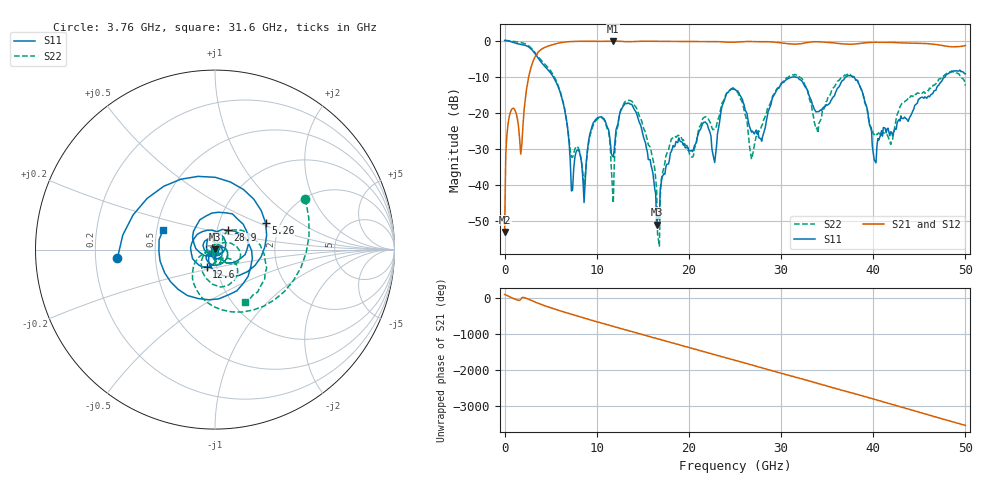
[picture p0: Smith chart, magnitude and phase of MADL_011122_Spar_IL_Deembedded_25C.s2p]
#	HZ	S	DB	R	50
!Frequency	S11 (dB)	S11-Ang	S21 Deemb (dB)	S21-Ang	S12 Deemb (dB)	S12-Ang	S22 (dB)	S22-Ang
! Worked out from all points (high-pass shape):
!   401 points, 10 MHz to 50 GHz, reference 50 ohm
!   highest |S21| = -0.15 dB at 11.8 GHz (marker M1); lowest = -53.1 dB at 10 MHz (marker M2)
!   |S21| within 3 dB of the highest: 3.681 GHz to end of sweep
!   lowest |S11| = -51.0 dB at 16.5 GHz (marker M3), VSWR 1.01, Z = 49.8 + j0.209 ohm
!   |S11| at or under -10 dB: 5.275 GHz to 37.1 GHz (31.83 GHz wide, 150 % of centre); 37.71 GHz to 47.82 GHz (10.1 GHz wide, 23.6 % of centre)
!   |S22| runs from -57.0 to 0.0 dB; largest |S21 - S12| = 0.017
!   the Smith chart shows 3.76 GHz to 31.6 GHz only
!   S11 on the Smith chart (normalised r, x): 3.76 GHz: 0.29, -0.04; 5.26 GHz: 1.67, +0.55; 12.6 GHz: 0.90, -0.17; 28.9 GHz: 1.12, +0.25; 31.6 GHz: 0.54, +0.13
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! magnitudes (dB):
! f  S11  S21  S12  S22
! 10 MHz  0.0  -53.1  -53.8  0.0
! 635 MHz  -0.3  -19.9  -19.9  -0.1
! 1.76 GHz  -1.1  -31.5  -31.5  -0.5
! 3.76 GHz  -5.3  -2.9  -2.9  -4.8
! 5.26 GHz  -9.9  -1.1  -1.1  -9.4
! 8.38 GHz  -34.2  -0.2  -0.2  -34.3
! 10.4 GHz  -21.2  -0.2  -0.2  -21.4
! 11.8 GHz  -32.3  -0.2  -0.1  -45.1
! 12.6 GHz  -19.5  -0.2  -0.2  -19.3
! 14.8 GHz  -23.7  -0.2  -0.2  -21.7
! 16.5 GHz  -51.0  -0.2  -0.2  -41.2
! 16.8 GHz  -49.7  -0.2  -0.2  -57.0
! 18.1 GHz  -30.8  -0.2  -0.2  -27.3
! 25.1 GHz  -13.8  -0.4  -0.4  -14.1
! 26.9 GHz  -25.1  -0.3  -0.3  -31.8
! 28.9 GHz  -17.8  -0.4  -0.4  -16.9
! 31.6 GHz  -10.2  -1.0  -1.0  -9.5
! 33.4 GHz  -17.8  -0.4  -0.3  -19.9
! 37.4 GHz  -9.8  -1.0  -1.0  -9.5
! 40.1 GHz  -33.0  -0.5  -0.5  -26.1
! 41.8 GHz  -26.4  -0.5  -0.5  -27.9
! 50 GHz  -9.2  -1.4  -1.4  -12.5
